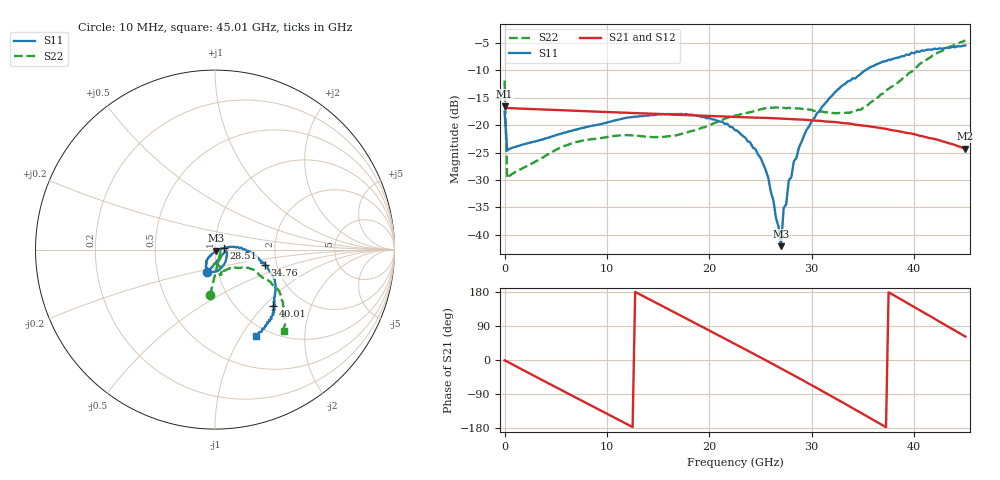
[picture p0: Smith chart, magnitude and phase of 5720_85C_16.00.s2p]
! Device:  ADRF5720
! Description: 0.5dB LSB GaAs MMIC 6-bit Digital Attenuator
! Frequency:  0.000009 -  40 GHz
! Ports:
!	RF1	= Port 1
!	RF2	= Port 2
! Vdd:  3.3 Volt
! Vss:  -3.3 Volt
! Control:  0/3.3 Volt
! State:  16.00 dB attenuation
! Data:  The device was measured using G-S-G Probes on a matrix board.
!  Data was collected using an calibrated 4 port network analyzer.
!  The reference plane for this measurement is at the launchers.
! Note:  Analog Devices supplies this data as a sample of measured data
!  for this product.  Your particular data for this product may vary.
!  Data was taken at 85 degrees C.
!  Analog Devices reserves the right to change this data at anytime.
# GHZ S DB R 45.0
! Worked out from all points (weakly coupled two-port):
!   181 points, 10 MHz to 45.01 GHz, reference 45 ohm
!   highest |S21| = -16.57 dB at 10 MHz (marker M1); lowest = -24.3 dB at 45.01 GHz (marker M2)
!   lowest |S11| = -42.1 dB at 27.01 GHz (marker M3), VSWR 1.02, Z = 45.5 - j0.468 ohm
!   |S11| at or under -10 dB: start of sweep to 35.24 GHz
!   |S22| runs from -29.7 to -4.5 dB; largest |S21 - S12| = 0.00073
!   S11 on the Smith chart (normalised r, x): 10 MHz: 0.89, -0.23; 28.51 GHz: 1.10, +0.02; 34.76 GHz: 1.73, -0.33; 40.01 GHz: 1.44, -1.13; 45.01 GHz: 0.86, -1.16
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0.01  -17.55 -108.4  -16.57 -1.1  -16.56 -1.1  -11.87 -96.1
0.26  -24.57 -8.9  -16.88 -3.9  -16.87 -3.9  -29.69 -15.4
4.26  -22.31 -33.0  -17.17 -61.2  -17.16 -61.1  -25.31 -55.6
7.76  -20.47 -56.6  -17.43 -110.4  -17.42 -110.3  -22.76 -80.0
15.26  -18.05 -94.9  -17.96 144.4  -17.95 144.5  -22.15 -89.5
20.01  -18.67 -113.3  -18.31 77.6  -18.29 77.8  -20.01 -74.2
22.76  -21.03 -122.3  -18.51 38.7  -18.49 38.9  -18.15 -73.2
24.51  -24.38 -127.7  -18.62 13.8  -18.61 14.1  -17.36 -75.5
25.51  -28.21 -123.4  -18.67 -0.6  -18.66 -0.3  -16.89 -76.8
26.26  -33.71 -116.0  -18.73 -11.5  -18.72 -11.2  -16.82 -76.6
27.01  -42.07 -40.7  -18.78 -22.4  -18.77 -22.2  -16.84 -76.8
27.26  -35.14 -12.9  -18.82 -26.2  -18.80 -25.9  -16.83 -77.5
27.51  -34.43 5.0  -18.85 -29.8  -18.83 -29.5  -16.92 -77.0
27.76  -30.09 5.1  -18.87 -33.4  -18.85 -33.1  -16.83 -77.8
28.51  -25.97 9.5  -18.95 -44.4  -18.93 -44.1  -16.96 -78.0
29.26  -21.84 10.9  -19.00 -55.5  -18.98 -55.2  -17.04 -77.2
30.26  -18.71 5.6  -19.15 -70.3  -19.13 -70.1  -17.43 -76.1
32.26  -14.01 -4.5  -19.42 -100.4  -19.41 -100.2  -17.83 -66.8
34.76  -10.69 -17.3  -19.99 -138.7  -19.98 -138.4  -17.22 -46.9
37.76  -8.06 -32.0  -20.89 174.9  -20.87 175.2  -13.02 -28.6
40.01  -6.91 -44.0  -21.65 139.7  -21.64 140.0  -9.74 -29.9
45.01  -5.46 -64.7  -24.31 61.9  -24.29 62.2  -4.55 -49.7
